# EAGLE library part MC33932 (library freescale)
5.0 A Throttle Control H-Bridge Auto generated by make-symbol-device-package-bsdl.ulp Rev. 33 Source: http://www.freescale.com/files/analog/doc/data_sheet/MC33932.pdf?fpsp=1
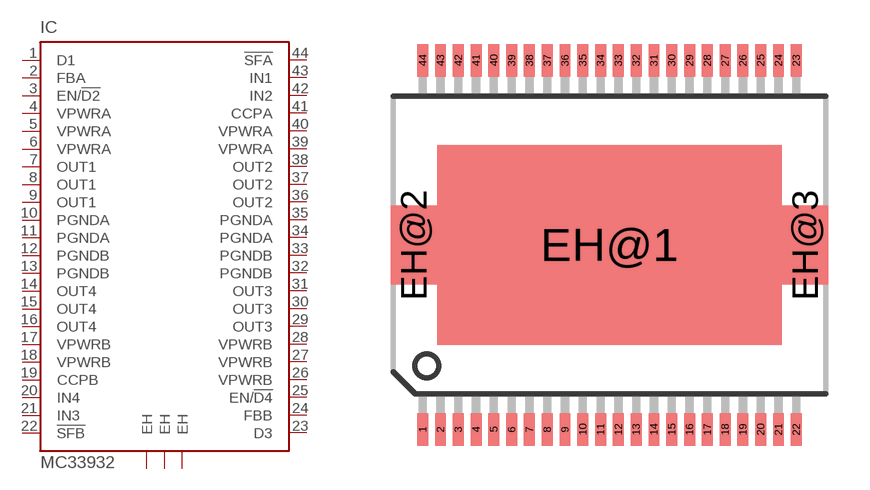
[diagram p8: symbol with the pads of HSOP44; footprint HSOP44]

Designator prefix IC

## MC33932 (MPN: MC33932VW; OC_FARNELL: 1701639; OC_NEWARK: 67P3304)  [HSOP44]
1  D1  in
2  FBA  out
3  EN/!D2  in
4  VPWRA  in
5  VPWRA  in
6  VPWRA  in
7  OUT1  out
8  OUT1  pas
9  OUT1  pas
10  PGNDA  pwr
11  PGNDA  pwr
12  PGNDB  pwr
13  PGNDB  pwr
14  OUT4  out
15  OUT4  pas
16  OUT4  pas
17  VPWRB  in
18  VPWRB  in
19  CCPB  out
20  IN4  in
21  IN3  in
22  !SFB  oc
23  D3  in
24  FBB  out
25  EN/!D4  in
26  VPWRB  in
27  VPWRB  in
28  VPWRB  in
29  OUT3  out
30  OUT3  pas
31  OUT3  pas
32  PGNDB  pwr
33  PGNDB  pwr
34  PGNDA  pwr
35  PGNDA  pwr
36  OUT2  out
37  OUT2  pas
38  OUT2  pas
39  VPWRA  in
40  VPWRA  in
41  CCPA  out
42  IN2  in
43  IN1  in
44  !SFA  oc
EH@1  EH  pas
EH@2  EH  pas
EH@3  EH  pas

## Footprint HSOP44 (pad centres in mm)
44 LEAD HSOP W/PROTRUDING HEADSINK Source: http://www.freescale.com/files/shared/doc/package_info/98ARH98330A.pdf
smd 0.4 x 1.2: 1 -6.825,-6.75; 2 -6.175,-6.75; 3 -5.525,-6.75; 4 -4.875,-6.75; 5 -4.225,-6.75; 6 -3.575,-6.75; 7 -2.925,-6.75; 8 -2.275,-6.75; 9 -1.625,-6.75; 10 -0.975,-6.75; 11 -0.325,-6.75; 12 0.325,-6.75; 13 0.975,-6.75; 14 1.625,-6.75; 15 2.275,-6.75; 16 2.925,-6.75; 17 3.575,-6.75; 18 4.225,-6.75; 19 4.875,-6.75; 20 5.525,-6.75; 21 6.175,-6.75; 22 6.825,-6.75; 23 6.825,6.75; 24 6.175,6.75; 25 5.525,6.75; 26 4.875,6.75; 27 4.225,6.75; 28 3.575,6.75; 29 2.925,6.75; 30 2.275,6.75; 31 1.625,6.75; 32 0.975,6.75; 33 0.325,6.75; 34 -0.325,6.75; 35 -0.975,6.75; 36 -1.625,6.75; 37 -2.275,6.75; 38 -2.925,6.75; 39 -3.575,6.75; 40 -4.225,6.75; 41 -4.875,6.75; 42 -5.525,6.75; 43 -6.175,6.75; 44 -6.825,6.75
smd 12.6 x 7.3: EH@1 0,0
smd 1.7 x 2.9: EH@2 -7.15,0; EH@3 7.15,0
